FUNCTION_BLOCK FB_LN_IED_LD1_LEDGGIO7 EXTENDS FB_AcsiCommonLogicalNodeClass
VAR_INPUT
	NamPlt: FB_DO_IED_LD1_LEDGGIO7_NamPlt := (sClass:='LPL', bLinkResult:=THIS^.AddDataToContainer(ipData:=NamPlt));
	Beh: FB_DO_IED_LD1_LEDGGIO7_Beh := (sClass:='ENS', bLinkResult:=THIS^.AddDataToContainer(ipData:=Beh));
	Health: FB_DO_IED_LD1_LEDGGIO7_Health := (sClass:='ENS', bLinkResult:=THIS^.AddDataToContainer(ipData:=Health));
	Mod_: FB_DO_IED_LD1_LEDGGIO7_Mod := (sObjectName:='Mod', sClass:='ENC', bLinkResult:=THIS^.AddDataToContainer(ipData:=Mod_));
	SPCSO1: FB_DO_IED_LD1_LEDGGIO7_SPCSO1 := (sClass:='SPC', bLinkResult:=THIS^.AddDataToContainer(ipData:=SPCSO1));
END_VAR
VAR
END_VAR

END_FUNCTION_BLOCK
